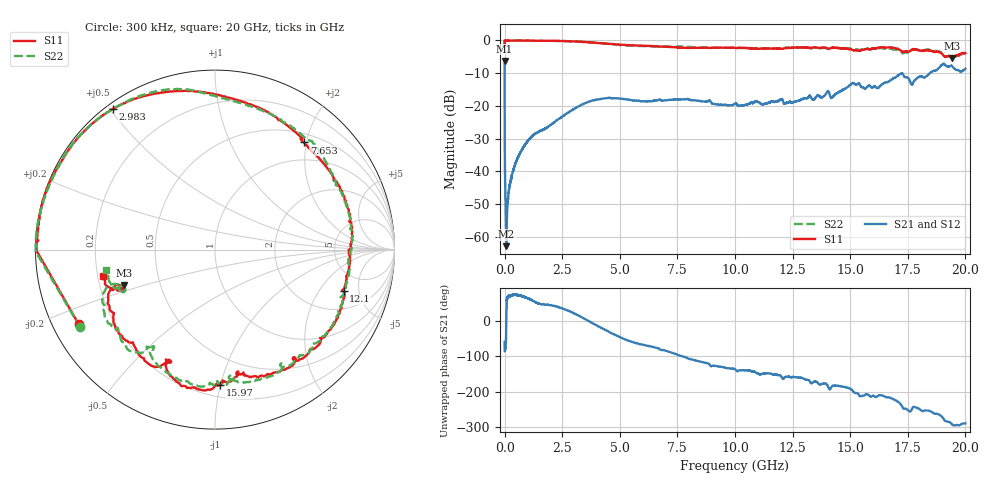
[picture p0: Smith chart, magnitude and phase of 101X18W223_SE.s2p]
!{101X18W223_SE}
!Johanson Technology Inc.
!www.johansontechnology.com
!Test Board Conditions:
!Substrate Type  RO4350B
!Substrate Thickness  21 mil
!Substrate Dk  3.66
!TL Type: GCPW
!TL Trace Width  40 mil
!TL Gap  20 mil
!PART MODE SINGLE ENDED (AKA BYPASS)
!DUT TOPOLOGY	SERIES-SHUNT
!Mounting Pad LxW  120x40 mil
! Created Wed Oct 27 11:09:46 2021
# hz S ma R 50
! 2 Port Network Data from SP1.SP block
! freq  magS11  angS11  magS21  angS21  magS12  angS12  magS22  angS22
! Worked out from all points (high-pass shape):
!   20001 points, 300 kHz to 20 GHz, reference 50 ohm
!   highest |S21| = -6.26 dB at 300 kHz (marker M1); lowest = -62.8 dB at 75.3 MHz (marker M2)
!   |S21| within 3 dB of the highest: 18.69 GHz to 19.74 GHz (1.043 GHz wide, 5.43 % of centre); 19.87 GHz to end of sweep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
!   lowest |S11| = -5.3 dB at 19.42 GHz (marker M3), VSWR 3.37, Z = 15.3 - j8.65 ohm
!   |S11| at or under -10 dB: nowhere
!   |S22| runs from -5.3 to 0.0 dB; largest |S21 - S12| = 0.012
!   S11 on the Smith chart (normalised r, x): 300 kHz: 0.08, -0.25; 2.983 GHz: 0.02, +0.51; 7.653 GHz: 0.65, +1.96; 12.1 GHz: 3.24, -3.46; 15.97 GHz: 0.29, -0.99; 20 GHz: 0.22, -0.11
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300000  0.866 -151.4  0.4865 -59.6  0.4882 -60.3  0.8675 -150.0
7.53e7  0.9938 178.7  0.0007228 8.9  0.0008626 8.9  0.9999 178.7
1.023e8  0.9922 178.2  0.001905 59.9  0.001955 60.8  0.9999 178.1
1.293e8  0.9938 177.6  0.003289 66.8  0.003254 64.4  0.9997 177.6
3.773e8  0.9927 173.0  0.01037 73.6  0.01047 72.7  0.9992 172.9
8.843e8  0.9974 163.8  0.02547 67.0  0.02569 67.1  0.9939 163.5
2.9833e9  0.9685 125.9  0.08875 22.2  0.0892 22.2  0.9634 123.3
3.3343e9  0.953 119.1  0.1038 10.7  0.1042 10.6  0.9514 115.7
6.6673e9  0.8113 64.9  0.1225 -77.2  0.1226 -77.5  0.8118 62.9
7.6533e9  0.7766 50.3  0.1257 -99.0  0.1253 -98.8  0.8076 46.6
1.00003e10  0.7694 12.4  0.1089 -136.3  0.1095 -136.2  0.7667 9.3
1.21033e10  0.753 -17.9  0.1128 -163.6  0.1118 -163.7  0.7573 -20.5
1.33343e10  0.7736 -40.1  0.1302 -176.0  0.1305 -175.4  0.761 -44.0
1.42323e10  0.7767 -56.3  0.1382 176.4  0.139 176.8  0.77 -62.5
1.51063e10  0.7162 -76.9  0.2255 162.3  0.2246 161.8  0.7296 -81.9
1.59703e10  0.7538 -88.0  0.1901 148.4  0.191 148.3  0.7519 -90.1
1.66673e10  0.7826 -100.2  0.2359 143.9  0.234 146.1  0.7495 -106.0
1.72123e10  0.6946 -113.1  0.3137 123.0  0.3163 124.1  0.6672 -122.7
1.76963e10  0.735 -117.1  0.2131 113.7  0.2157 113.3  0.7236 -128.0
1.84493e10  0.7055 -141.8  0.3136 105.6  0.317 105.5  0.7161 -149.3
1.94173e10  0.5426 -158.4  0.4068 68.1  0.4052 68.2  0.5431 -157.5
2e10  0.6383 -166.7  0.3703 70.8  0.3698 70.1  0.6157 -169.9
